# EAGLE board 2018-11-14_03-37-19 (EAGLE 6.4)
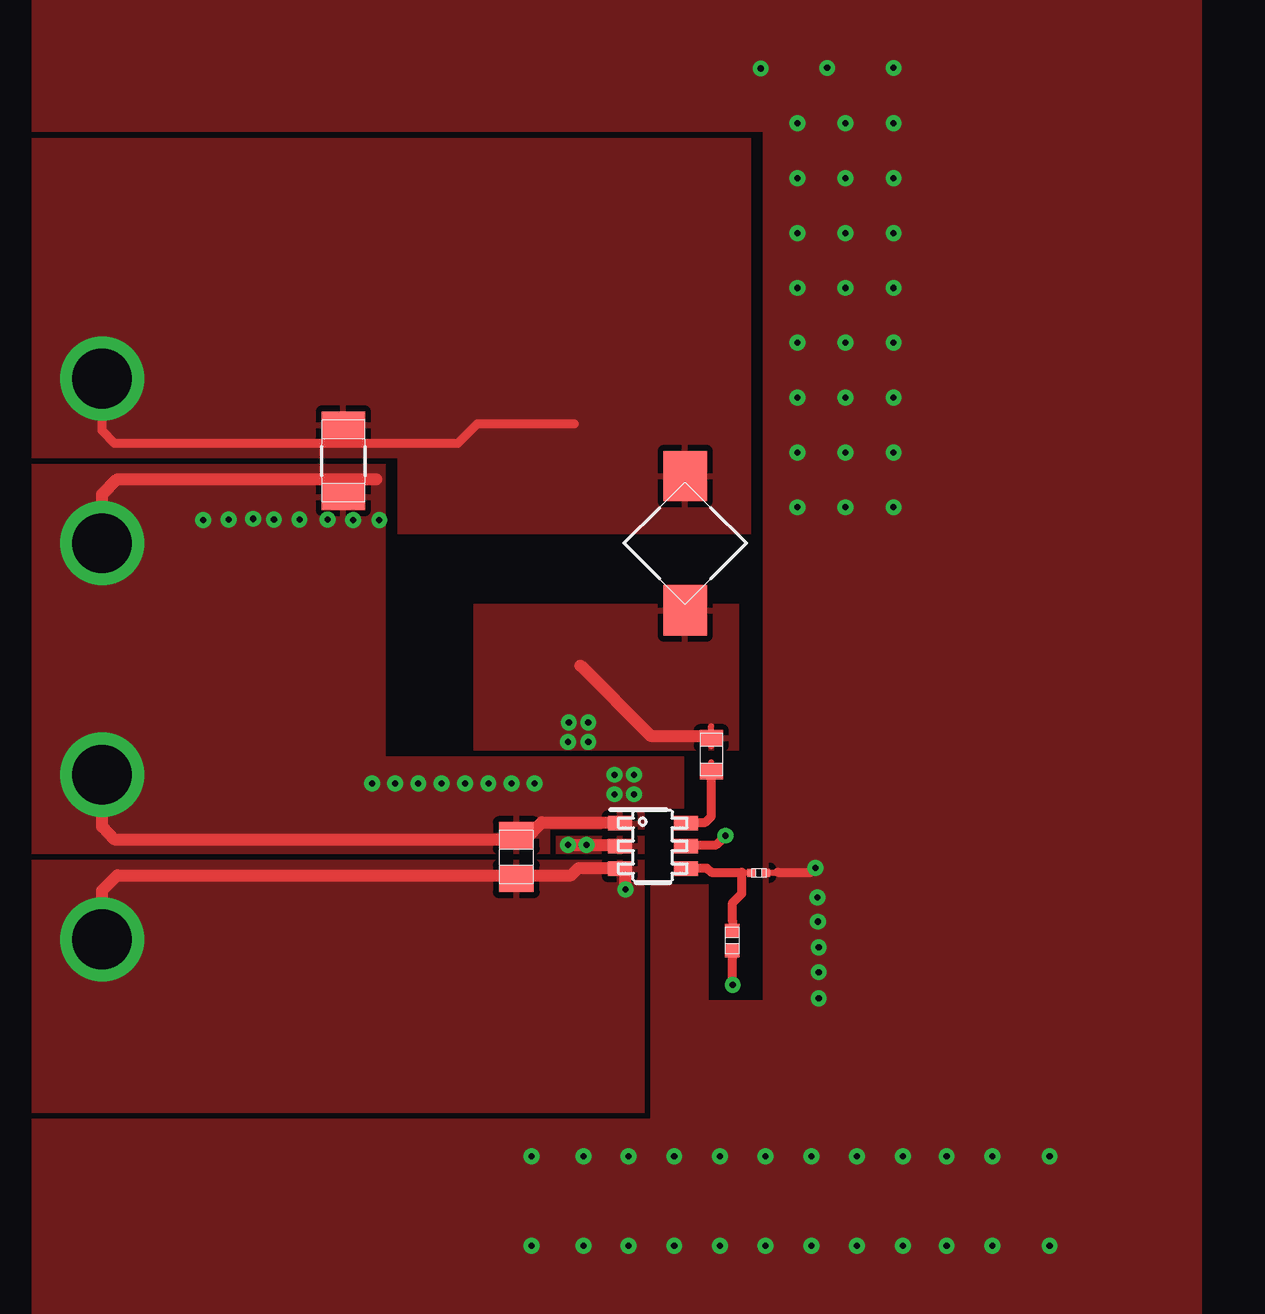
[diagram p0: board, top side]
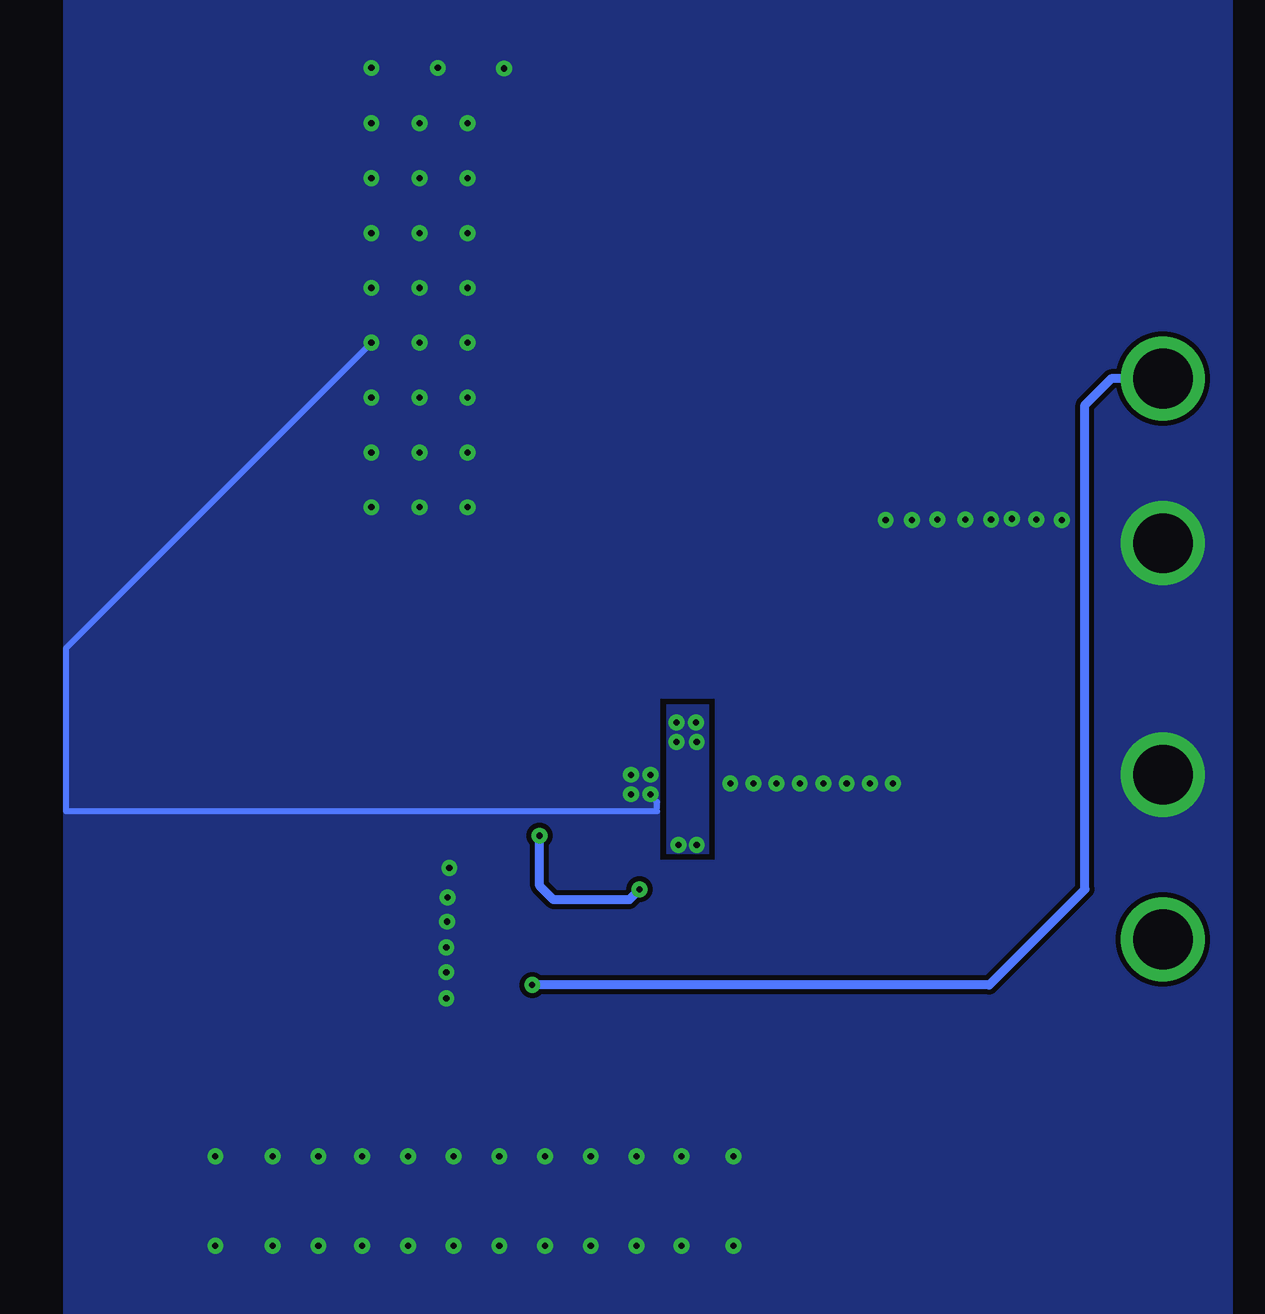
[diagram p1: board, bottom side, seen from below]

No outline drawn. Coordinates in mm, seen from the top.
Copper layers ((1*2)+(15*16)): TOP / INTERNAL1 / layer 15 / BOTTOM

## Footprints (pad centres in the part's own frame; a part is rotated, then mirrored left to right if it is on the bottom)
0603 = smd 0.66 x 0.965: 1 -0.699,0; 2 0.699,0
0805 = smd 1.118 x 1.448: 1 -0.902,0; 2 0.902,0
1206 = smd 1.118 x 1.803: 1 -1.499,0; 2 1.499,0
TP-1502 = drill 0.813 round: 1 0,0
CDPH4D19F = smd 2.095 x 1.803: 1 -2.8,0; 2 2.8,0
0201 = smd 0.356 x 0.33: 1 -0.292,0; 2 0.292,0
0402 = smd 0.559 x 0.61: 1 -0.419,0; 2 0.419,0
DDC0006A = smd 1 x 0.6: 1 -1.375,0.95; 2 -1.375,0; 3 -1.375,-0.95; 4 1.375,-0.95; 5 1.375,0; 6 1.375,0.95

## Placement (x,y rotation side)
Cbst  [0603]  54.74,51.77 270 top
Cin  [0805]  46.61,47.5 90 top
Cout  [1206]  39.4,64.01 270 top
GND  [TP-1502]  29.34,60.53 90 top
GND1  [TP-1502]  29.34,50.9 90 top
L1  [CDPH4D19F]  53.64,60.58 90 top
Rfbb  [0201]  56.72,46.84 0 top
Rfbt  [0402]  55.6,44.02 90 top
U1  [DDC0006A]  52.3,47.96 0 top
VIN  [TP-1502]  29.34,44.02 90 top
VOUT  [TP-1502]  29.34,67.44 90 top

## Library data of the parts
Cbst = ultra-librarian; RefDes: Cbst; Type: C0603C104Z3VACTU
Cin = ultra-librarian; RefDes: Cin; Type: C2012X5R1V226M125AC
Cout = ultra-librarian; RefDes: Cout; Type: C3216X5R1E476M160AC
GND = ultra-librarian; RefDes: GND; Type: TP-1502
GND1 = ultra-librarian; RefDes: GND1; Type: TP-1502
L1 = ultra-librarian; RefDes: L1; Type: CDPH4D19FNP-4R7MC
Rfbb = ultra-librarian; RefDes: Rfbb; Type: RC0201FR-0710KL
Rfbt = ultra-librarian; RefDes: Rfbt; Type: CRCW040261K9FKED
U1 = ultra-librarian; RefDes: U1; Type: TPS561201DDCR
VIN = ultra-librarian; RefDes: VIN; Type: TP-1502
VOUT = ultra-librarian; RefDes: VOUT; Type: TP-1502

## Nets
0: Cin.2 Cout.2 GND1.1 GND.1 Rfbb.2 U1.1
2: Cbst.1 L1.1 U1.2
3: Rfbb.1 Rfbt.2 U1.4
4: Cout.1 L1.2 Rfbt.1 VOUT.1
5: Cbst.2 U1.6
9: Cin.1 U1.3 U1.5 VIN.1

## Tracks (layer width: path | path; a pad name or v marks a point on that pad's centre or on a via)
0  (via drill 0.25 pad 0.61, 2.49 pad 3.48)
  TOP 0.254: 57.07,46.85 57.91,46.85
  TOP 0.381: 57.51,46.86 58.9,46.86 v59.08,47.04
  TOP 0.508: 40.77,63.25 29.97,63.25 29.34,62.61 v29.34,60.58 | 51.16,48.95 47.68,48.95 46.99,48.23 29.84,48.23 29.34,48.77 v29.34,50.93
  BOTTOM 0.254: v62.33,68.94 75.06,56.21 75.06,49.4 50.42,49.4 50.42,49.78 50.7,50.06 v50.7,50.11
  other vias: 40.59,50.57 68.83,31.29 68.83,35.03 47.24,31.29 47.24,35.03 64.54,31.29 66.45,31.29 66.45,35.03 64.54,35.03 51.51,50.93 50.7,50.93 47.37,50.57 46.41,50.57 45.44,50.57 44.48,50.57 43.48,50.57 42.52,50.57 41.55,50.57 35.64,61.59 34.62,61.57 33.55,61.54 40.89,61.54 39.8,61.54 38.73,61.57 37.57,61.57 36.5,61.57 51.51,50.11 49.4,35.03 51.28,35.03 53.19,35.03 55.09,35.03 57,35.03 58.9,35.03 60.81,35.03 62.71,35.03 59.16,45.82 59.18,44.81 59.21,43.74 59.21,42.7 59.21,41.61 58.32,73.51 58.32,71.22 58.32,68.94 58.32,66.65 60.33,73.51 60.33,71.22 60.33,68.94 62.33,73.51 62.33,71.22 62.33,66.65 62.71,31.29 60.81,31.29 58.9,31.29 57,31.29 55.09,31.29 53.19,31.29 51.28,31.29 49.4,31.29 62.33,75.79 62.33,78.08 62.33,80.39 60.33,75.79 60.33,78.08 59.56,80.39 58.32,75.79 58.32,78.08 56.79,80.37 62.33,62.08 62.33,64.36 60.33,64.36 58.32,62.08 58.32,64.36 60.33,62.08 60.33,66.65
  pour TOP: 26.42,47.62 48.01,47.62 48.01,48.64 51.94,48.64 51.94,49.53 53.59,49.53 53.59,51.69 41.15,51.69 41.15,63.88 26.42,63.88
  pour TOP: 26.42,36.58 26.42,26.29 75.18,26.29 75.18,85.47 26.42,85.47 26.42,77.72 56.9,77.72 56.9,41.53 54.61,41.53 54.61,46.35 52.2,46.35 52.2,36.58
  pour BOTTOM (rank 6): 26.42,26.29 75.18,26.29 75.18,49.4 50.29,49.4 50.29,47.37 48.01,47.37 48.01,54.1 50.29,54.1 50.29,49.53 75.18,49.53 75.18,85.47 26.42,85.47
2  (via drill 0.25 pad 0.61)
  TOP 0.254: 54.72,52.12 54.72,52.96
  TOP 0.508: 49.28,55.47 52.2,52.55 54.74,52.55 | v48.77,48.01 51.16,48.01 | 51.16,48.01
  other vias: 49.53,48.01 48.79,53.11 49.61,53.11 49.61,52.3 48.77,52.3
  pour TOP (rank 2): 55.88,58.04 44.83,58.04 44.83,51.94 55.88,51.94
  pour TOP (rank 5): 51.94,48.39 51.94,47.62 48.26,47.62 48.26,48.39
  pour BOTTOM: 48.26,47.62 48.26,53.85 50.04,53.85 50.04,47.62
3
  TOP 0.254: 55.58,46.85 56.41,46.85 | 55.61,44.37 55.61,45.21
  TOP 0.381: 53.49,47.04 54.53,47.04 54.74,46.86 56.01,46.86 56.01,45.97 55.63,45.59 55.63,44.81
4  (via drill 0.25 pad 0.61, 2.49 pad 3.48)
  TOP 0.254: 55.61,42.88 55.61,43.71
  TOP 0.381: 49.02,65.56 44.98,65.56 44.17,64.75 40.26,64.75 29.84,64.75 29.34,65.28 VOUT.1 | v55.63,42.16 | v55.63,42.16 55.63,43.31
  BOTTOM 0.381: VOUT.1 31.5,67.44 32.59,66.34 32.59,46.15 36.58,42.16 v55.63,42.16
  other vias: 29.34,67.44
  pour TOP (rank 4): 56.39,60.96 41.66,60.96 41.66,64.14 26.42,64.14 26.42,77.47 56.39,77.47
5
  TOP 0.254: 54.72,50.62 54.72,51.46
  TOP 0.381: 53.49,48.95 54.48,48.95 54.74,49.2 54.74,51.05
9  (via drill 0.25 pad 0.61, 2.49 pad 3.48)
  TOP 0.381: v55.32,48.39 54.94,48.01 53.49,48.01
  TOP 0.508: v51.16,46.15 51.16,47.04 49.2,47.04 48.9,46.74 46.99,46.74 29.97,46.74 29.34,46.1 v29.34,44.07
  BOTTOM 0.381: v55.32,48.39 55.32,46.3 54.74,45.72 51.59,45.72 v51.16,46.15
  pour TOP (rank 3): 26.42,47.37 51.94,47.37 51.94,36.83 26.42,36.83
